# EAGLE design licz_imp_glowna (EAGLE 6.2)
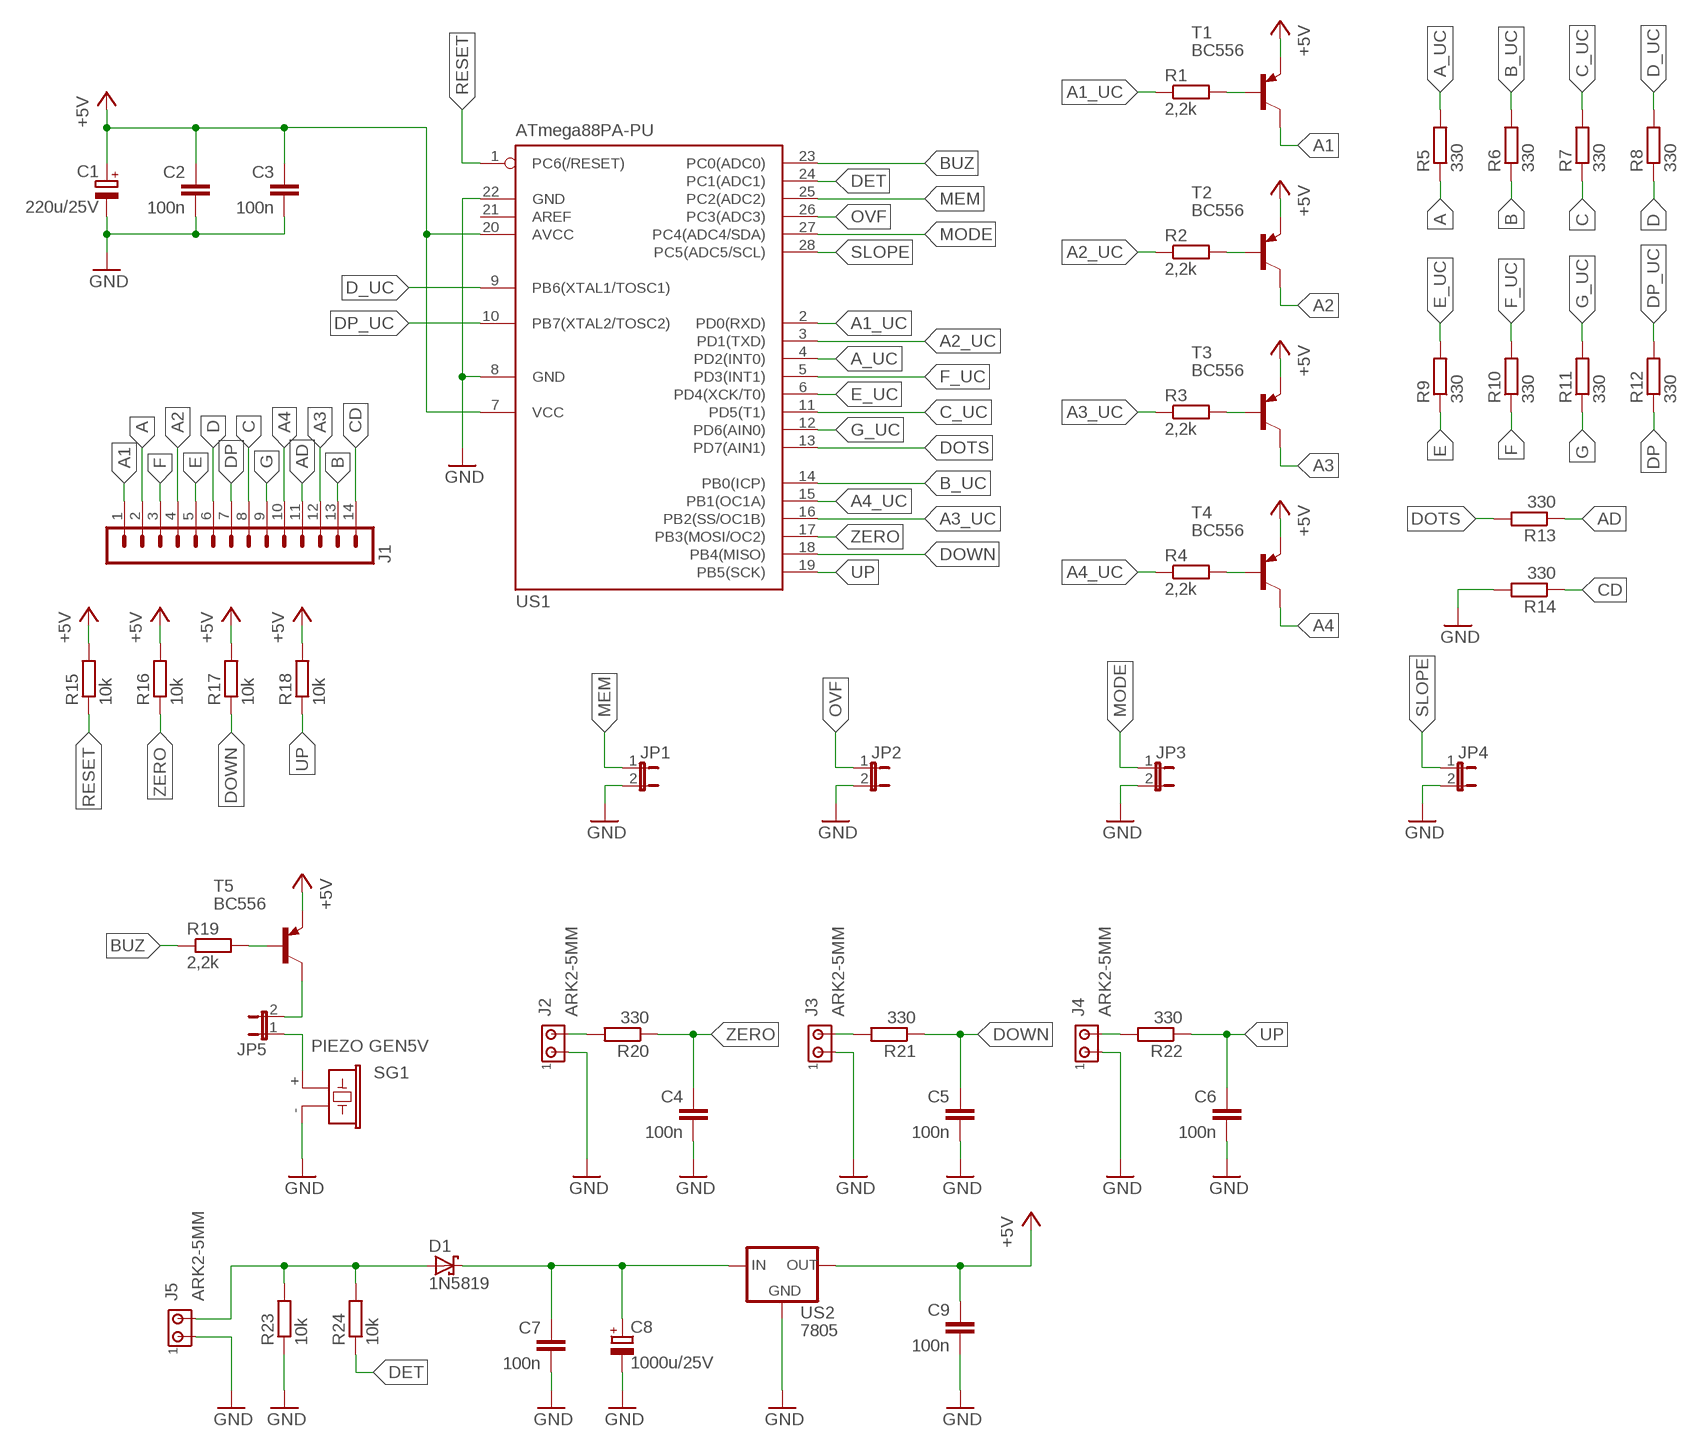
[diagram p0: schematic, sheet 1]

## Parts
C1  220u/25V  CPOL-EUE2.5-7  [E2,5-7]
C2  100n  C-EU050-025X075  [C050-025X075]
C3  100n  C-EU050-025X075  [C050-025X075]
C4  100n  C-EU050-025X075  [C050-025X075]
C5  100n  C-EU050-025X075  [C050-025X075]
C6  100n  C-EU050-025X075  [C050-025X075]
C7  100n  C-EU050-025X075  [C050-025X075]
C8  1000u/25V  CPOL-EUE5-10.5  [E5-10,5]
C9  100n  C-EU050-025X075  [C050-025X075]
D1  1N5819  1N5819-T  [DO41-7.6]
J1  MA14-1  [MA14-1]
J2  ARK2-5MM  [2PIN-5MM]
J3  ARK2-5MM  [2PIN-5MM]
J4  ARK2-5MM  [2PIN-5MM]
J5  ARK2-5MM  [2PIN-5MM]
JP1  JP1E  [JP1]
JP2  JP1E  [JP1]
JP3  JP1E  [JP1]
JP4  JP1E  [JP1]
JP5  JP1E  [JP1]
R1  2,2k  R-EU_0207/7  [0207/7]
R2  2,2k  R-EU_0207/7  [0207/7]
R3  2,2k  R-EU_0207/7  [0207/7]
R4  2,2k  R-EU_0207/7  [0207/7]
R5  330  R-EU_0207/7  [0207/7]
R6  330  R-EU_0207/7  [0207/7]
R7  330  R-EU_0207/7  [0207/7]
R8  330  R-EU_0207/7  [0207/7]
R9  330  R-EU_0207/7  [0207/7]
R10  330  R-EU_0207/7  [0207/7]
R11  330  R-EU_0207/7  [0207/7]
R12  330  R-EU_0207/7  [0207/7]
R13  330  R-EU_0207/7  [0207/7]
R14  330  R-EU_0207/7  [0207/7]
R15  10k  R-EU_0207/7  [0207/7]
R16  10k  R-EU_0207/7  [0207/7]
R17  10k  R-EU_0207/7  [0207/7]
R18  10k  R-EU_0207/7  [0207/7]
R19  2,2k  R-EU_0207/7  [0207/7]
R20  330  R-EU_0207/7  [0207/7]
R21  330  R-EU_0207/7  [0207/7]
R22  330  R-EU_0207/7  [0207/7]
R23  10k  R-EU_0207/7  [0207/7]
R24  10k  R-EU_0207/7  [0207/7]
SG1  PIEZO GEN5V  F/CM12P  [F/CM12P]
T1  BC556  [TO92-EBC]
T2  BC556  [TO92-EBC]
T3  BC556  [TO92-EBC]
T4  BC556  [TO92-EBC]
T5  BC556  [TO92-EBC]
US1  ATmega88PA-PU  MEGA8-P  [DIL28-3]
US2  7805  78XXS  [78XXS]

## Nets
+5V: C1.+ C2.1 C3.1 C9.1 R15.2 R16.2 R17.2 R18.2 T1.E T2.E T3.E T4.E T5.E US1.7(VCC) US1.20(AVCC) US2.OUT
A: J1.2 R5.1
A1: J1.1 T1.C
A1_UC: R1.1 US1.2(PD0(RXD))
A2: J1.4 T2.C
A2_UC: R2.1 US1.3(PD1(TXD))
A3: J1.12 T3.C
A3_UC: R3.1 US1.16(PB2(SS/OC1B))
A4: J1.10 T4.C
A4_UC: R4.1 US1.15(PB1(OC1A))
A_UC: R5.2 US1.4(PD2(INT0))
AD: J1.11 R13.1
B: J1.13 R6.1
B_UC: R6.2 US1.14(PB0(ICP))
BUZ: R19.1 US1.23(PC0(ADC0))
C: J1.8 R7.1
C_UC: R7.2 US1.11(PD5(T1))
CD: J1.14 R14.1
D: J1.6 R8.1
D_UC: R8.2 US1.9(PB6(XTAL1/TOSC1))
DET: R24.1 US1.24(PC1(ADC1))
DOTS: R13.2 US1.13(PD7(AIN1))
DOWN: C5.1 R17.1 R21.1 US1.18(PB4(MISO))
DP: J1.7 R12.1
DP_UC: R12.2 US1.10(PB7(XTAL2/TOSC2))
E: J1.5 R9.1
E_UC: R9.2 US1.6(PD4(XCK/T0))
F: J1.3 R10.1
F_UC: R10.2 US1.5(PD3(INT1))
G: J1.9 R11.1
G_UC: R11.2 US1.12(PD6(AIN0))
GND: C1.- C2.2 C3.2 C4.2 C5.2 C6.2 C7.2 C8.- C9.2 J2.P$1 J3.P$1 J4.P$1 J5.P$1 JP1.2 JP2.2 JP3.2 JP4.2 R14.2 R23.1 SG1.- US1.8(GND) US1.22(GND) US2.GND
MEM: JP1.1 US1.25(PC2(ADC2))
MODE: JP3.1 US1.27(PC4(ADC4/SDA))
N$1: R1.2 T1.B
N$2: R19.2 T5.B
N$3: JP5.1 SG1.+
N$4: JP5.2 T5.C
N$5: J2.P$2 R20.2
N$6: J3.P$2 R21.2
N$7: J4.P$2 R22.2
N$8: D1.A J5.P$2 R23.2 R24.2
N$9: C7.1 C8.+ D1.C US2.IN
N$11: R2.2 T2.B
N$12: R3.2 T3.B
N$13: R4.2 T4.B
OVF: JP2.1 US1.26(PC3(ADC3))
RESET: R15.1 US1.1(PC6(/RESET))
SLOPE: JP4.1 US1.28(PC5(ADC5/SCL))
UP: C6.1 R18.1 R22.1 US1.19(PB5(SCK))
ZERO: C4.1 R16.1 R20.1 US1.17(PB3(MOSI/OC2))
Unconnected: US1.21(AREF)

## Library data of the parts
C1 C8 = rcl:CPOL-EU: POLARIZED CAPACITOR, European symbol
C2-C7 C9 = rcl:C-EU: CAPACITOR, European symbol
D1 = diode:1N581*: 1.0A SCHOTTKY BARRIER RECTIFIER
J1 = zlacza_futrzak:MA14-1: PIN HEADER; OC_FARNELL: unknown; OC_NEWARK: unknown
J2-J5 = zlacza_futrzak:ARK2: ARK 2
JP1-JP5 = jumper:JP1E: JUMPER
R1-R24 = rcl:R-EU_: RESISTOR, European symbol
SG1 = buzzer:F/CM12P: BUZZER; OC_FARNELL: unknown; OC_NEWARK: unknown
T1-T5 = transistor-pnp:BC556*: PNP Transistror
US1 = atmel:MEGA8-P: MICROCONTROLLER 8 Kbytes FLASH, 1 kbytes SRAM, 512 bytes EEPROM, USART, 4-channel 10 bit ADC, 2-channel 8 bit ADC Pin compatible with Atmega48, ATMega88, ATMega168 Source: avr.lbr; OC_FARNELL: unknown; OC_NEWARK: unknown
US2 = v-reg:78XXS: VOLTAGE REGULATOR

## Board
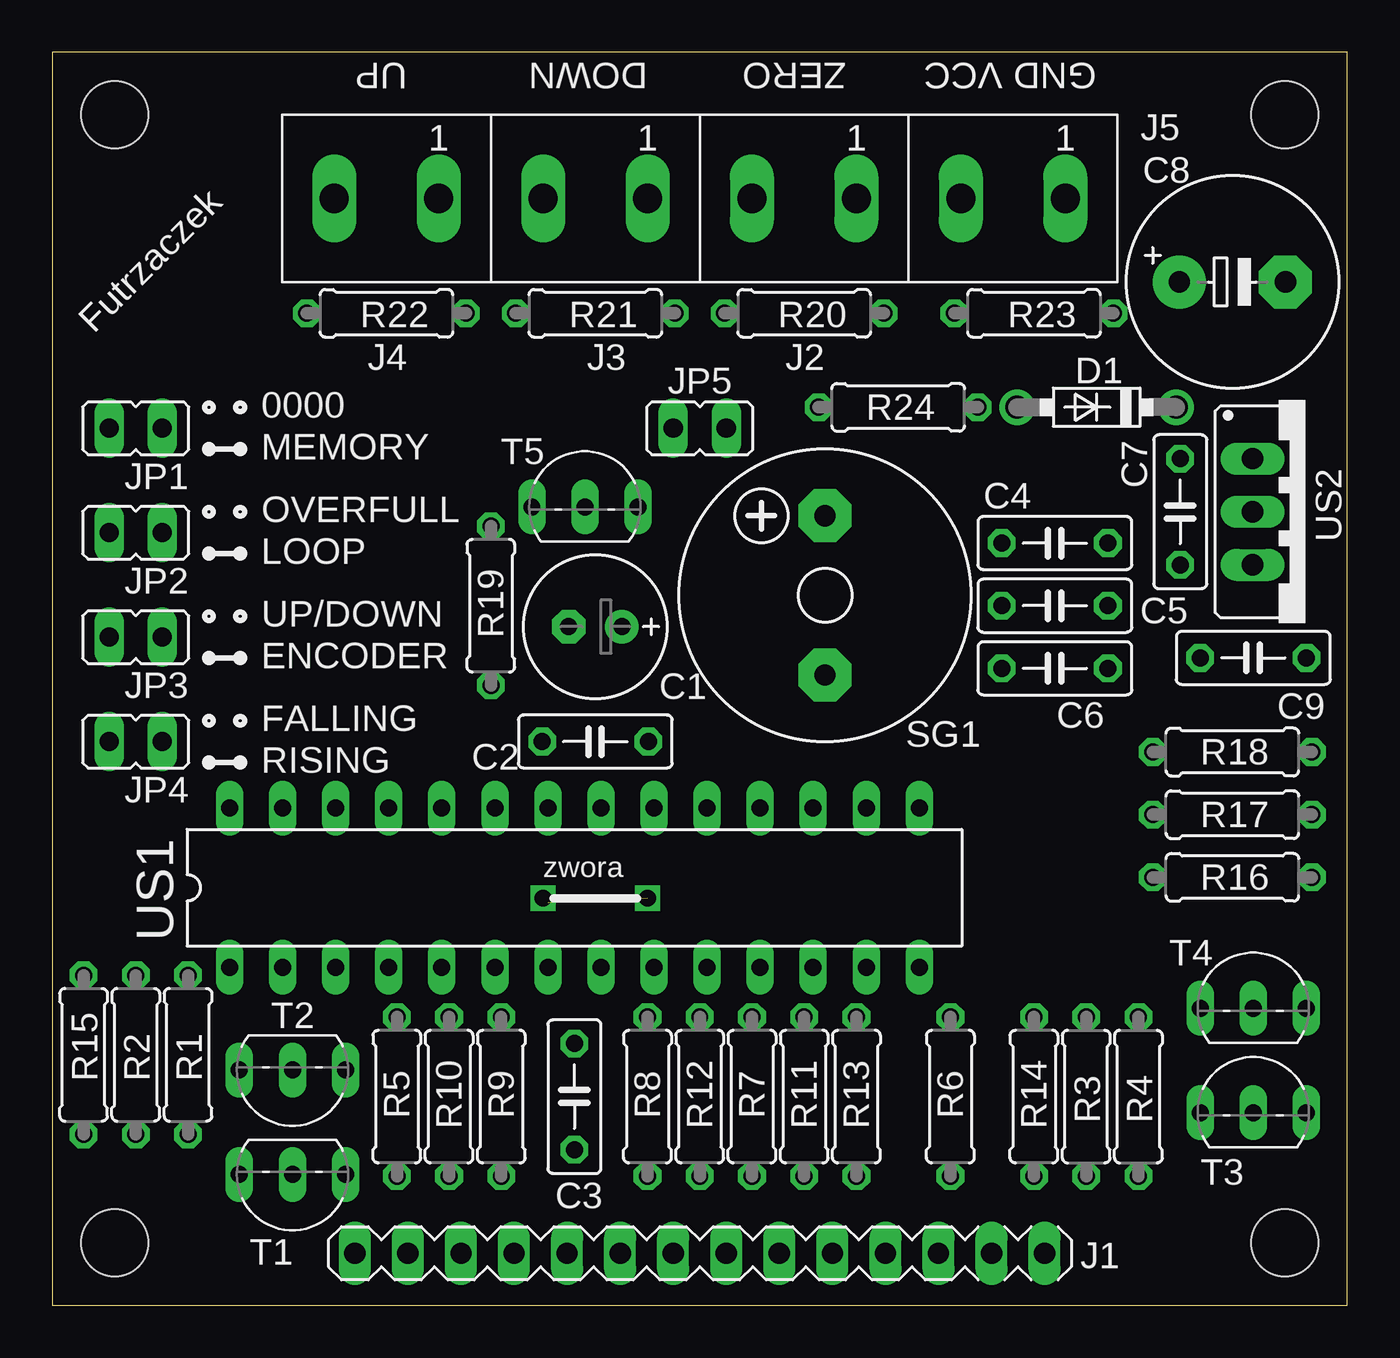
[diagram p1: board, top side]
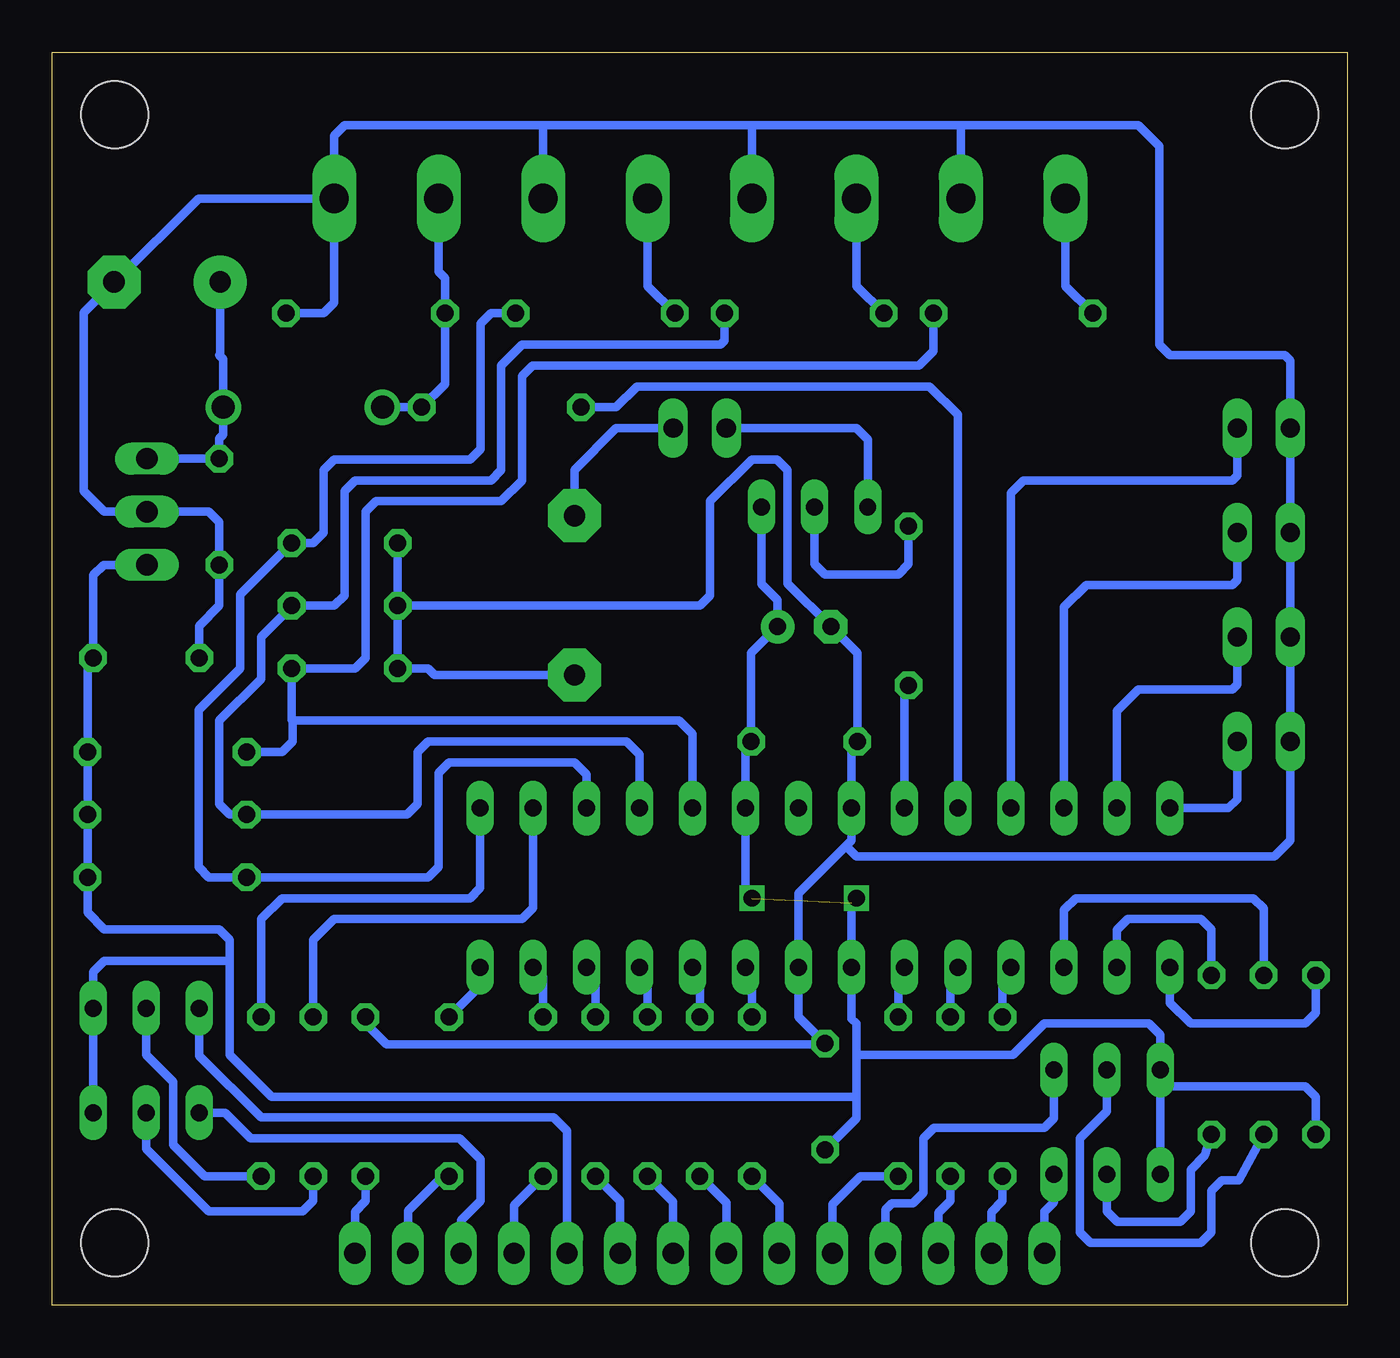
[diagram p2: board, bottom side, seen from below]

Size 62 x 60 mm. Coordinates in mm from the lower left corner, seen from the top.
Outline: 0,0 62,0 62,60 0,60 0,0
Copper layers (1*16): Top 0.035mm / dielectric 1.5mm / Bottom 0.035mm
Design rules: minimum track width 10mil, minimum drill 24mil, track to track 8mil, track to pad 8mil, pad to pad 8mil, via to via 8mil, smd to smd 8mil, copper to edge 15mil, drill to drill 8mil, minimum pad ring 10mil, minimum via ring 8mil, stop-mask expansion 4mil, vias tented up to drill 0mil, thermal gap 10mil
Holes 3.2 mm at 3,3 59,3 3,57 59,57

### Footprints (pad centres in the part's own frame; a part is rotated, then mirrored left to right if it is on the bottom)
E2,5-7 = drill 0.813 pad 1.6: + -1.27,0 | drill 0.813 pad 1.6 octagon: - 1.27,0
C050-025X075 = drill 0.813 octagon: 1 -2.54,0; 2 2.54,0
E5-10,5 = drill 1.016 pad 2.54: + -2.54,0 | drill 1.016 pad 2.54 octagon: - 2.54,0
DO41-7.6 = drill 1.1 pad 1.7: A 3.81,0; C -3.81,0
MA14-1 = drill 1.016 long: 1 -16.51,0; 2 -13.97,0; 3 -11.43,0; 4 -8.89,0; 5 -6.35,0; 6 -3.81,0; 7 -1.27,0; 8 1.27,0; 9 3.81,0; 10 6.35,0; 11 8.89,0; 12 11.43,0; 13 13.97,0; 14 16.51,0
2PIN-5MM = drill 1.4 long: P$1 -2.5,0; P$2 2.5,0
JP1 = drill 0.914 long: 1 0,-1.27; 2 0,1.27
0207/7 = drill 0.813 octagon: 1 -3.81,0; 2 3.81,0
F/CM12P = drill 1.016 pad 2.54 octagon: + 3.81,0; - -3.81,0
TO92-EBC = drill 0.813 long: B 0,-1.27; C -2.54,-1.27; E 2.54,-1.27
DIL28-3 = drill 0.813 long: 1 -16.51,-3.81; 2 -13.97,-3.81; 3 -11.43,-3.81; 4 -8.89,-3.81; 5 -6.35,-3.81; 6 -3.81,-3.81; 7 -1.27,-3.81; 8 1.27,-3.81; 9 3.81,-3.81; 10 6.35,-3.81; 11 8.89,-3.81; 12 11.43,-3.81; 13 13.97,-3.81; 14 16.51,-3.81; 15 16.51,3.81; 16 13.97,3.81; 17 11.43,3.81; 18 8.89,3.81; 19 6.35,3.81; 20 3.81,3.81; 21 1.27,3.81; 22 -1.27,3.81; 23 -3.81,3.81; 24 -6.35,3.81; 25 -8.89,3.81; 26 -11.43,3.81; 27 -13.97,3.81; 28 -16.51,3.81
78XXS = drill 1.016 long: GND 0,-2.54; IN -2.54,-2.54; OUT 2.54,-2.54

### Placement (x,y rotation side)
C1  26,32.5 180 top
C2  26,27 180 top
C3  25,10 90 top
C4  48,36.5 180 top
C5  48,33.5 180 top
C6  48,30.5 180 top
C7  54,38 270 top
C8  56.5,49 0 top
C9  57.5,31 180 top
D1  50,43 180 top
J1  31,2.5 0 top
J2  36,53 180 top
J3  26,53 180 top
J4  16,53 180 top
J5  46,53 180 top
JP1  4,42 90 top
JP2  4,37 90 top
JP3  4,32 90 top
JP4  4,27 90 top
JP5  31,42 90 top
R1  6.5,12 270 top
R2  4,12 270 top
R3  49.5,10 270 top
R4  52,10 270 top
R5  16.5,10 90 top
R6  43,10 90 top
R7  33.5,10 90 top
R8  28.5,10 90 top
R9  21.5,10 90 top
R10  19,10 90 top
R11  36,10 90 top
R12  31,10 90 top
R13  38.5,10 90 top
R14  47,10 90 top
R15  1.5,12 270 top
R16  56.5,20.5 0 top
R17  56.5,23.5 0 top
R18  56.5,26.5 0 top
R19  21,33.5 90 top
R20  36,47.5 180 top
R21  26,47.5 180 top
R22  16,47.5 180 top
R23  47,47.5 180 top
R24  40.5,43 0 top
SG1  37,34 90 top
T1  11.5,5 180 top
T2  11.5,10 180 top
T3  57.5,10.5 0 top
T4  57.5,15.5 0 top
T5  25.5,39.5 0 top
US1  25,20 0 top
US2  60,38 270 top

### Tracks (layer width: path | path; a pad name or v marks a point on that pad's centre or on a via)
+5V  (via drill 0.8)  (1 unrouted)
  Bottom 0.406: T1.E 8.96,10.5 | 8.96,10.5 T2.E 8.96,12.96 9.5,13.5 14.5,13.5 16,12 23.5,12 | 23.5,12 23.5,13.5 23.73,13.73 US1.7 23.73,19.27 v23.5,19.5 | 23.5,12 23.5,10 | 23.5,10 23.5,8.96 C3.1 | R15.2 1.5,10 2,10.5 8.96,10.5 | T3.E T4.E 60.04,15.96 59.5,16.5 53.5,16.5 | 23.5,10 51.5,10 53.5,12 53.5,16.5 | v28.5,19.5 28.81,19.81 US1.20 28.81,26.73 C2.1 28.54,31.23 C1.+ 27.27,33.77 28.04,34.54 T5.E | 53.5,16.5 53.5,17.5 54,18 59.5,18 60.31,18.81 R16.2 R17.2 R18.2 60.31,30.73 C9.1 60.04,34.96 59.54,35.46 US2.OUT
A
  Bottom 0.406: J1.2 17.03,4.47 16.5,5 R5.1
A1
  Bottom 0.406: J1.1 14.49,4.49 | 14.49,4.49 14.5,4.5 | T1.C 14.04,4.94 14.49,4.49
A1_UC
  Bottom 0.406: R1.1 6.5,18 7,18.5 10.5,18.5 11.03,17.97 US1.2
A2
  Bottom 0.406: T2.C 14.04,8.96 14.5,8.5 19.8,8.5 20.3,8 20.3,5.4 20.8,4.9 21.8,4.9 22.11,4.59 J1.4
A2_UC
  Bottom 0.406: R2.1 4,19 4.5,19.5 13,19.5 13.57,18.93 US1.3
A3
  Bottom 0.406: J1.12 42.43,4.07 41.5,5 41.5,7 42.5,8 52.5,8 53.73,9.23 T3.C
A3_UC
  Bottom 0.406: US1.16 38.97,19.03 39.5,18.5 48.5,18.5 49.5,17.5 R3.1
A4
  Bottom 0.406: T4.C 54.96,11.96 52,9 38,9 37.35,8.35 J1.10
A4_UC
  Bottom 0.406: US1.15 41.51,19.99 42,19.5 51,19.5 52,18.5 R4.1
A_UC
  Bottom 0.406: R5.2 16.5,15.8 US1.4
AD
  Bottom 0.406: J1.11 39.89,4.8 R13.1
B
  Bottom 0.406: J1.13 44.97,4.53 43.31,6.19 R6.1
B_UC
  Bottom 0.406: US1.14 41.51,15.3 R6.2
BUZ
  Bottom 0.406: US1.23 21.19,29.5 R19.1
C
  Bottom 0.406: J1.8 32.27,4.96 R7.1
C_UC
  Bottom 0.406: R7.2 33.5,15.8 US1.11
CD
  Bottom 0.406: J1.14 47.51,4.49 47,5 R14.1
D
  Bottom 0.406: J1.6 27.19,4.88 R8.1
D_UC
  Bottom 0.406: R8.2 28.5,15.88 US1.9
DET
  Bottom 0.406: US1.24 18.65,42.65 20,44 34,44 35,43 R24.1
DOTS
  Bottom 0.406: R13.2 38.5,15.72 US1.13
DOWN
  Bottom 0.406: US1.18 33.89,26.39 34.5,27 44,27 44.5,26.5 44.5,24 45,23.5 R17.1 53.5,23.5 54,24 54,28 52,30 52,32 50.54,33.46 C5.1 48.5,33.5 48,34 48,39 47.5,39.5 41,39.5 40.5,40 40.5,45 39.5,46 30,46 29.81,46.19 R21.1
DP
  Bottom 0.406: J1.7 29.73,4.92 R12.1
DP_UC
  Bottom 0.406: R12.2 31,15.84 US1.10
E
  Bottom 0.406: J1.5 24.65,4.85 23.31,6.19 R9.1
E_UC
  Bottom 0.406: R9.2 21.5,15.88 US1.6
F
  Bottom 0.406: J1.3 19.57,4.43 19,5 R10.1
F_UC
  Bottom 0.406: R10.2 19,15.84 US1.5
G
  Bottom 0.406: J1.9 34.81,5 R11.1
G_UC
  Bottom 0.406: R11.2 36,15.76 US1.12
GND
  Bottom 0.406: R14.2 47,13.5 46,12.5 25.04,12.5 C3.2 26.27,13.81 US1.8 26.27,19.73 24,22 | 24,22 23.73,22.27 US1.22 23.73,26.73 C2.2 23.46,31.23 C1.- 26.8,34.57 26.8,40 27.3,40.5 28.5,40.5 30.5,38.5 30.5,34 31,33.5 C5.2 | 24,22 23.5,21.5 3.5,21.5 2.73,22.27 JP4.2 JP3.2 JP2.2 JP1.2 2.73,45.23 3,45.5 8.5,45.5 9,46 9,55.5 10,56.5 18.5,56.5 | SG1.- 43.69,30.19 44,30.5 C6.2 C5.2 | C5.2 C4.2 | J5.P$1 48.5,48 49,47.5 R23.1 | C9.2 54.96,32.54 54,33.5 C7.2 54,37.5 54.5,38 US2.GND 59.5,38 60.5,39 60.5,47.54 C8.- 59,49 55,53 J5.P$1 | J5.P$1 48.5,56 48,56.5 38.5,56.5 | 38.5,56.5 28.5,56.5 | 28.5,56.5 18.5,56.5 | J4.P$1 18.5,56.5 | J3.P$1 28.5,56.5 | J2.P$1 38.5,56.5
MEM
  Bottom 0.406: JP1.1 5.27,39.73 5.5,39.5 15.5,39.5 16.11,38.89 US1.25
MODE
  Bottom 0.406: JP3.1 5.27,29.73 5.5,29.5 10,29.5 11.03,28.47 US1.27
N$1
  Bottom 0.406: T1.B 11.5,4.5 11,4 8,4 7.5,4.5 7.5,6.5 6.81,7.19 R1.2
N$2
  Bottom 0.406: T5.B 25.5,35.5 25,35 21.5,35 21,35.5 R19.2
N$3
  Bottom 0.406: JP5.1 35,42 37,40 SG1.+
N$4
  Bottom 0.406: T5.C 22.96,41.46 23.5,42 JP5.2
N$5
  Bottom 0.406: J2.P$2 33.5,48.81 R20.2
N$6
  Bottom 0.406: J3.P$2 23.5,48.81 R21.2
N$7
  Bottom 0.406: J4.P$2 13.5,48.81 R22.2
N$8
  Bottom 0.406: J5.P$2 43.5,49.5 43.19,49.19 R23.2 43.19,44.12 R24.2 D1.A
N$9
  Bottom 0.406: C8.+ 53.96,45.54 54,45.5 53.81,45.31 D1.C 53.81,41.69 54,41.5 C7.1 US2.IN
N$11
  Bottom 0.406: T2.B 11.5,9.3 12.8,8 12.8,3.5 12.3,3 7,3 6.5,3.5 6.5,5.5 6,6 5.19,6 R2.2
N$12
  Bottom 0.406: R3.2 49.5,5 50,4.5 54.5,4.5 57.5,7.5 T3.B
N$13
  Bottom 0.406: R4.2 54.69,6.19 56.2,7.7 56.2,10.7 57.5,12 T4.B
OVF
  Bottom 0.406: JP2.1 5.27,34.73 5.5,34.5 12.5,34.5 13.57,33.43 US1.26
RESET
  Bottom 0.406: US1.1 8.49,14.49 7.5,13.5 2,13.5 1.5,14 R15.1
SLOPE
  Bottom 0.406: US1.28 5.69,23.81 5.27,24.23 JP4.1
UP
  Bottom 0.406: US1.19 31.35,27.35 32,28 50.5,28 | 50.5,28 50.54,28.04 C6.1 47.5,30.5 47,31 47,38 46.5,38.5 40.5,38.5 39.5,39.5 39.5,44.5 39,45 20.5,45 19.81,45.69 R22.1 | 50.5,28 50.5,27 51,26.5 R18.1
ZERO
  Bottom 0.406: US1.17 36.43,25.43 37,26 43,26 43.5,25.5 43.5,21 44,20.5 R16.1 54.5,20.5 55,21 55,28.5 53,30.5 53,34.04 C4.1 49.5,36.5 49,37 49,40 48.5,40.5 42,40.5 41.5,41 41.5,47 41,47.5 R20.1

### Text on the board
tPlace: UP | DOWN | ZERO | GND VCC | Futrzaczek | 0000 | MEMORY | OVERFULL | LOOP | UP/DOWN | ENCODER | FALLING | RISING | zwora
